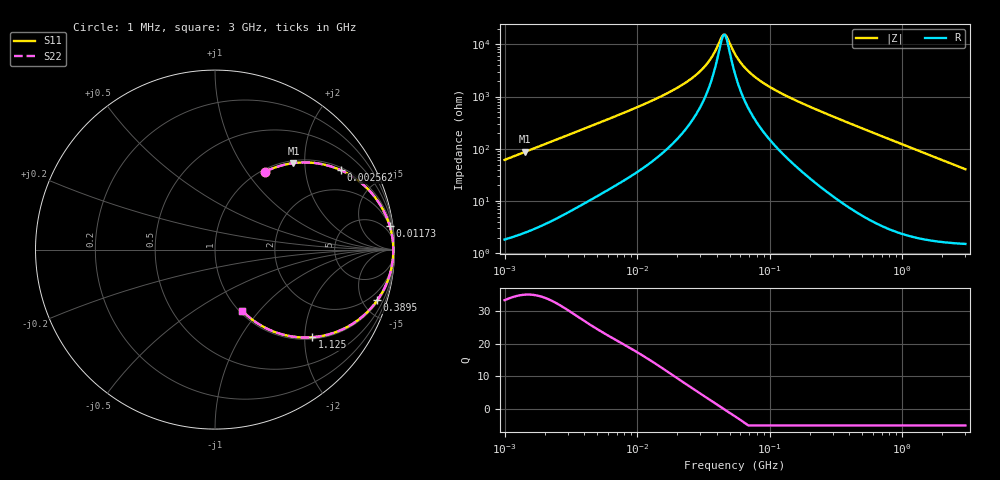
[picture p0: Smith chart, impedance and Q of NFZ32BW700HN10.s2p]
! NFZ32BW700HN10
# Hz S RI R 50
!Freq.(Hz) S11(Real) S11(Imag) S21(Real) S21(Imag) S12(Real) S12(Imag) S22(Real) S22(Imag)
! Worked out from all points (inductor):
!   401 points, 1 MHz to 3 GHz, reference 50 ohm
!   read as one part in series: L = 9.74 uH near 1.041 MHz
!   highest Q = 35.1 at 1.434 MHz (marker M1), where L = 9.74 uH
!   self-resonance near 44.84 MHz
!   S11 on the Smith chart (normalised r, x): 1 MHz: 1.04, +1.23; 2.562 MHz: 1.10, +3.12; 11.73 MHz: 2, +15; 389.5 MHz: 1.16, -6.35; 1.125 GHz: 1.04, -2.17; 3 GHz: 1.03, -0.81
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1000000  0.2797 0.4341  0.7203 -0.4341  0.7203 -0.4341  0.2797 0.4341
1433740  0.4368 0.4819  0.5632 -0.4819  0.5632 -0.4819  0.4368 0.4819
2561897  0.7036 0.4413  0.2964 -0.4413  0.2964 -0.4413  0.7036 0.4413
3823119  0.8354 0.3531  0.1646 -0.3531  0.1646 -0.3531  0.8354 0.3531
6305767  0.9275 0.2377  0.0725 -0.2377  0.0725 -0.2377  0.9275 0.2377
1.172775e7  0.9744 0.1293  0.0256 -0.1293  0.0256 -0.1293  0.9744 0.1293
1.461624e7  0.9819 0.1007  0.0181 -0.1007  0.0181 -0.1007  0.9819 0.1007
2.225279e7  0.9898 0.0567  0.0102 -0.0567  0.0102 -0.0567  0.9898 0.0567
3.00453e7  0.9924 0.0312  0.00763 -0.0312  0.00763 -0.0312  0.9924 0.0312
3.597591e7  0.9932 0.0173  0.00683 -0.0173  0.00683 -0.0173  0.9932 0.0173
4.483659e7  0.9936 0.001  0.00644 -0.001  0.00644 -0.001  0.9936 0.001
4.761141e7  0.9936 -0.00342  0.00643 0.00342  0.00643 0.00342  0.9936 -0.00342
5.477226e7  0.9934 -0.0138  0.00658 0.0138  0.00658 0.0138  0.9934 -0.0138
6.558369e7  0.9929 -0.0276  0.00713 0.0276  0.00713 0.0276  0.9929 -0.0276
8.507507e7  0.9912 -0.0491  0.00879 0.0491  0.00879 0.0491  0.9912 -0.0491
1.244416e8  0.986 -0.0866  0.014 0.0866  0.014 0.0866  0.986 -0.0866
2.094008e8  0.9678 -0.1573  0.0322 0.1573  0.0322 0.1573  0.9678 -0.1573
3.894533e8  0.9041 -0.2825  0.0959 0.2825  0.0959 0.2825  0.9041 -0.2825
8.005644e8  0.6968 -0.4503  0.3032 0.4503  0.3032 0.4503  0.6968 -0.4503
1.125055e9  0.5403 -0.4885  0.4597 0.4885  0.4597 0.4885  0.5403 -0.4885
1.931433e9  0.2904 -0.441  0.7096 0.441  0.7096 0.441  0.2904 -0.441
3e9  0.1511 -0.34  0.8489 0.34  0.8489 0.34  0.1511 -0.34
